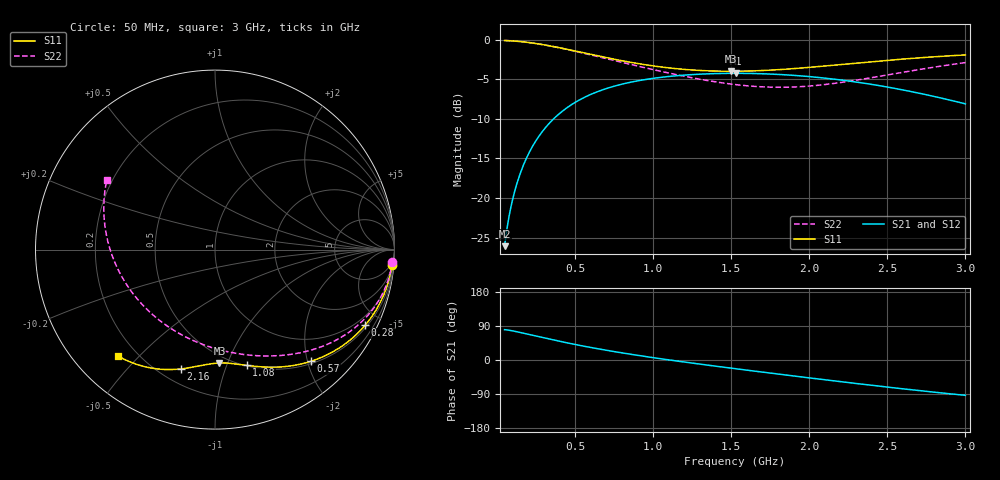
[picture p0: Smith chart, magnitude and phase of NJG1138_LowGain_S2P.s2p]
! NJG1138 Low gain mode
# hz S ri R 50
! 2 Port Network Data from SP1.SP block
! freq  reS11  imS11  reS21  imS21  reS12  imS12  reS22  imS22
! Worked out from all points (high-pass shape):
!   296 points, 50 MHz to 3 GHz, reference 50 ohm
!   highest |S21| = -4.24 dB at 1.53 GHz (marker M1); lowest = -26.1 dB at 50 MHz (marker M2)
!   |S21| within 3 dB of the highest: 564.9 MHz to 2.817 GHz (2.252 GHz wide, 133 % of centre)
!   lowest |S11| = -4.0 dB at 1.5 GHz (marker M3), VSWR 4.44, Z = 22.2 - j46.8 ohm
!   |S11| at or under -10 dB: nowhere
!   |S22| runs from -6.0 to -0.1 dB; largest |S21 - S12| = 6.7e-08
!   S11 on the Smith chart (normalised r, x): 50 MHz: 3, -22; 280 MHz: 0.60, -4.13; 570 MHz: 0.54, -2.07; 1.08 GHz: 0.51, -1.18; 2.16 GHz: 0.28, -0.72; 3 GHz: 0.13, -0.43
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5e7  0.9854 -0.0865  0.00856 0.0489  0.00856 0.0489  0.9877 -0.0688
7e7  0.98 -0.1198  0.0129 0.0673  0.0129 0.0673  0.9835 -0.0951
9e7  0.9729 -0.1527  0.0185 0.0854  0.0185 0.0854  0.9782 -0.1213
1.4e8  0.9482 -0.2322  0.0379 0.1283  0.0379 0.1283  0.9594 -0.1848
2e8  0.907 -0.3201  0.0704 0.1738  0.0704 0.1738  0.9278 -0.2562
2.8e8  0.8368 -0.421  0.1255 0.2209  0.1255 0.2209  0.8731 -0.3402
4e8  0.7135 -0.5336  0.2214 0.2594  0.2214 0.2594  0.774 -0.4398
5.5e8  0.5564 -0.6149  0.3411 0.2574  0.3411 0.2574  0.6392 -0.5219
5.7e8  0.5365 -0.6217  0.3559 0.2536  0.3559 0.2536  0.6211 -0.5299
8e8  0.3392 -0.655  0.4956 0.1698  0.4956 0.1698  0.4218 -0.5838
1.04e9  0.1948 -0.647  0.5758 0.039  0.5758 0.039  0.2319 -0.591
1.08e9  0.1757 -0.6446  0.5831 0.0156  0.5831 0.0156  0.2017 -0.5888
1.28e9  0.0953 -0.6344  0.5962 -0.1024  0.5962 -0.1024  0.0542 -0.5653
1.5e9  0.0247 -0.6318  0.5709 -0.2253  0.5709 -0.2253  -0.1022 -0.5149
1.53e9  0.0157 -0.6322  0.5646 -0.2409  0.5646 -0.2409  -0.123 -0.5059
1.77e9  -0.0558 -0.642  0.4933 -0.3522  0.4933 -0.3522  -0.2826 -0.4142
2.02e9  -0.1381 -0.6575  0.3887 -0.4344  0.3887 -0.4344  -0.4273 -0.2816
2.16e9  -0.1898 -0.6647  0.3223 -0.4626  0.3223 -0.4626  -0.4937 -0.193
2.34e9  -0.262 -0.6683  0.2349 -0.4793  0.2349 -0.4793  -0.5594 -0.0685
2.51e9  -0.3344 -0.6631  0.1555 -0.476  0.1555 -0.476  -0.5993 0.0546
2.74e9  -0.434 -0.6402  0.0605 -0.4476  0.0605 -0.4476  -0.6195 0.2194
3e9  -0.541 -0.5923  -0.0225 -0.393  -0.0225 -0.393  -0.6026 0.3896
